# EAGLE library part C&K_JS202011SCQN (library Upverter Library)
Sub-miniature slide switch DPDT
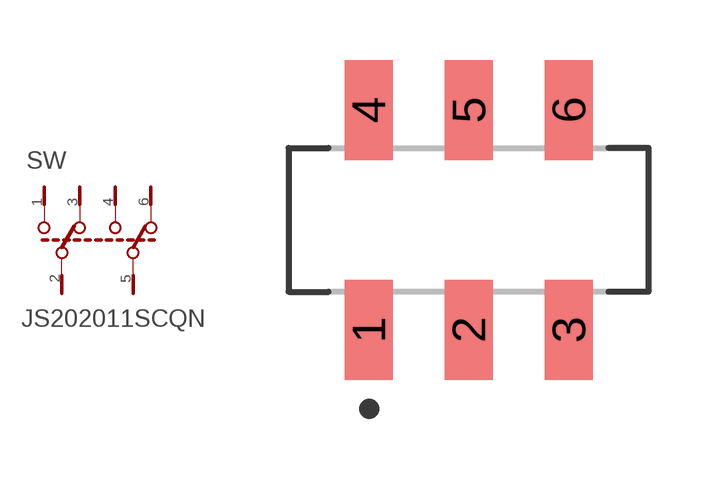
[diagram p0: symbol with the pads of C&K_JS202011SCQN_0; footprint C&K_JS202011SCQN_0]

Designator prefix SW

## C&K_JS202011SCQNC&K_JS202011SCQN_0_0 (Actuator_Type: Standard; Circuit: DPDT; Contact_Rating_@_Voltage: 0.3A @ 6VDC; MF: C&K; MPN: JS202011SCQN; Orientation: Vertical; Termination_Style: Gull Wing; centroid_not_specified: No; datasheet: https://upverter.com/datasheet/c27b63fdc98daa115a91c8449f599d1446fad1e5.pdf; digikey_description: SWITCH SLIDE DPDT 300MA 6V; digikey_part_number: 401-2002-1-ND; imported_from: PartsBot; lead_free: yes; mounting_type: Surface Mount; mouser_part_number: 611-JS202011SCQN; num_pins: 6; octopart_part_number: 94a55dc393914b62; package: SW_DPDT_SMT_9MM0_3MM6; prefix: SW; rohs: yes; temperature_range_high: +85°C; temperature_range_low: -40°C; voltage: 6V)  [C&K_JS202011SCQN_0]
1  1
2  2
3  3
4  4
5  5
6  6

## Footprint C&K_JS202011SCQN_0 (pad centres in mm)
Sub-miniature slide switch DPDT
smd 1.2 x 2.5: 1 -2.5,-2.75; 2 0,-2.75; 3 2.5,-2.75; 4 -2.5,2.75; 5 0,2.75; 6 2.5,2.75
